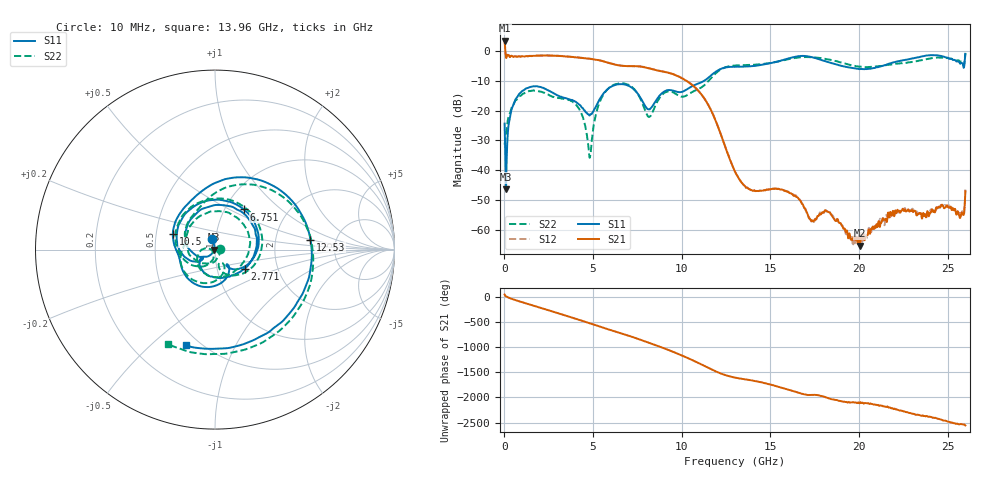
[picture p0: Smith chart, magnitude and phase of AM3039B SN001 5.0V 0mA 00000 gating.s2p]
!Agilent Technologies,E8364B,MY43040894,A.07.50.67
!Agilent E8364B: A.07.50.67
!Date: Tuesday, June 28, 2016 08:03:20
!Correction: S11(Full 2 Port(1,2))
!S21(Full 2 Port(1,2))
!S12(Full 2 Port(1,2))
!S22(Full 2 Port(1,2))
!S2P File: Measurements: S11, S21, S12, S22:
# Hz S  dB  R 50
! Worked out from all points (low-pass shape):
!   1601 points, 10 MHz to 26 GHz, reference 50 ohm
!   highest |S21| = 3.53 dB at 10 MHz (marker M1); lowest = -65.4 dB at 20.05 GHz (marker M2)
!   |S21| within 3 dB of the highest: start of sweep to 44.95 MHz
!   lowest |S11| = -46.4 dB at 91.22 MHz (marker M3), VSWR 1.01, Z = 49.5 + j0.00805 ohm
!   |S11| at or under -10 dB: start of sweep to 11.26 GHz
!   |S22| runs from -35.8 to -0.6 dB; largest |S21 - S12| = 0.024
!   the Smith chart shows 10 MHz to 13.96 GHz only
!   S11 on the Smith chart (normalised r, x): 10 MHz: 0.96, +0.11; 2.771 GHz: 1.36, -0.30; 6.751 GHz: 1.22, +0.59; 10.5 GHz: 0.61, +0.11; 12.53 GHz: 3.21, +0.51; 13.96 GHz: 0.42, -0.65
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1e7  -24.36 108.5  3.53 40.4  3.58 41.3  -31.43 12.5
9.121875e7  -46.40 179.0  -2.18 4.6  -2.08 4.6  -28.10 -59.5
7.24725e8  -15.43 162.1  -1.92 -81.5  -1.87 -81.3  -16.10 174.7
1.585644e9  -11.89 72.5  -1.60 -174.4  -1.56 -174.3  -13.29 76.3
2.771438e9  -14.13 -32.5  -1.55 57.4  -1.47 57.6  -15.39 -31.1
4.347081e9  -18.86 -138.5  -2.29 -116.9  -2.25 -116.8  -21.03 -169.7
5.565362e9  -14.44 -175.0  -3.42 103.2  -3.35 103.3  -14.81 -162.3
6.751156e9  -11.20 54.3  -5.01 -28.1  -4.96 -28.0  -10.87 46.6
8.684162e9  -15.47 -67.2  -6.58 95.7  -6.52 95.9  -16.40 -76.9
1.050346e10  -12.04 159.9  -10.95 -165.8  -10.90 -165.8  -14.05 146.7
1.253393e10  -5.43 6.0  -33.51 -127.4  -33.42 -127.6  -5.31 1.0
1.3005e10  -5.27 -33.9  -40.49 -168.5  -40.43 -168.7  -4.83 -40.7
1.396338e10  -5.08 -107.0  -46.77 134.4  -46.66 134.9  -4.63 -116.3
1.61238e10  -2.30 85.1  -47.72 -58.8  -47.75 -60.0  -2.56 82.5
1.734208e10  -2.04 -30.0  -56.96 -150.7  -57.59 -152.9  -2.05 -20.4
1.873904e10  -4.50 -147.7  -56.90 107.4  -56.41 104.9  -3.40 -136.1
2.005479e10  -6.03 118.6  -65.40 54.1  -65.00 65.9  -5.22 128.5
2.167916e10  -4.22 11.3  -55.32 -45.4  -55.48 -49.2  -4.62 17.3
2.307612e10  -2.39 -93.4  -53.97 -167.5  -53.45 -172.7  -3.58 -83.4
2.414821e10  -1.33 179.6  -53.53 116.2  -53.45 118.8  -2.32 -165.2
2.513908e10  -2.53 94.9  -52.36 28.7  -52.74 25.5  -2.51 111.6
2.6e10  -1.03 -26.7  -47.09 -37.8  -46.52 -38.5  -0.59 1.4
